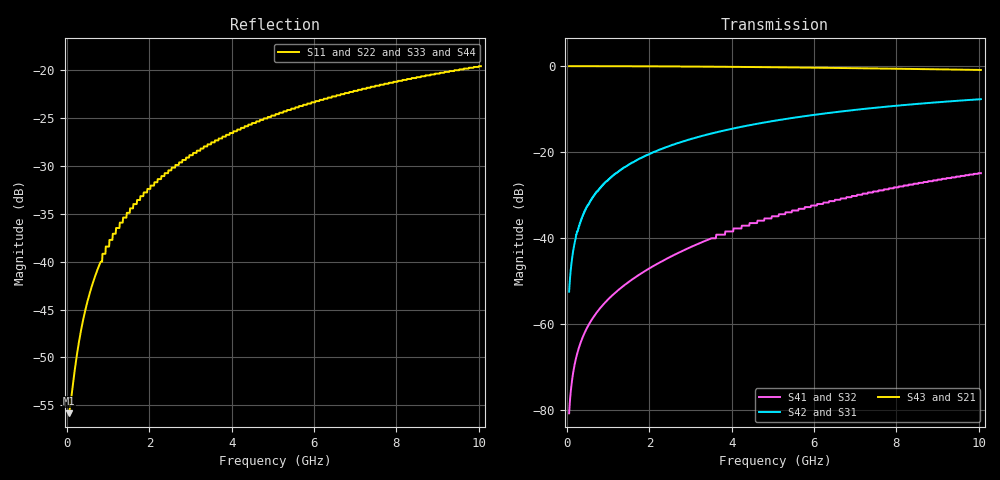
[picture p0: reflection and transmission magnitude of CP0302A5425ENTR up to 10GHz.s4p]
!	AVX THIN FILM OPERATION
!	CP0302A5425ENTR HIGH DIRECTIVITY  COUPLER
!	P/N's CP0302A5425ENTR
! 	18 August 2013
# MHZ S MA R 50
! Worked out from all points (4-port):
!   1000 points, 50 MHz to 10.05 GHz, reference 50 ohm
!   strongest paths, dB at 50 MHz, 2.553 GHz, 5.055 GHz, 7.558 GHz, 10.05 GHz:
!     S43: 0.0, -0.1, -0.3, -0.6, -0.9
!     S21: 0.0, -0.1, -0.3, -0.6, -0.9
!     S42: -52.4, -18.3, -12.7, -9.6, -7.7
!     S31: -52.4, -18.3, -12.7, -9.6, -7.7
!     S41: -80.7, -44.1, -34.9, -29.1, -24.9
!     S32: -80.7, -44.1, -34.9, -29.1, -24.9
!   lowest |S11| = -55.8 dB at 50 MHz (marker M1), VSWR 1.00, Z = 50.2 + j0.0605 ohm
!   |S11| at or under -10 dB: start of sweep to end of sweep
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50  0.001616 21.9  0.998 -0.2  0.002398 89.8  9.252e-05 90.6
    0.998 -0.2  0.001616 21.9  9.252e-05 90.6  0.002398 89.8
    0.002398 89.8  9.252e-05 90.6  0.001616 21.9  0.998 -0.2
    9.252e-05 90.6  0.002398 89.8  0.998 -0.2  0.001616 21.9
240.19  0.003279 62.1  0.998 -0.9  0.012 89.2  0.0004459 93.4
        0.998 -0.9  0.003279 62.1  0.0004459 93.4  0.012 89.2
        0.012 89.2  0.0004459 93.4  0.003279 62.1  0.998 -0.9
        0.0004459 93.4  0.012 89.2  0.998 -0.9  0.003279 62.1
590.541  0.007322 76.4  0.998 -2.1  0.028 87.9  0.001114 98.3
         0.998 -2.1  0.007322 76.4  0.001114 98.3  0.028 87.9
         0.028 87.9  0.001114 98.3  0.007322 76.4  0.998 -2.1
         0.001114 98.3  0.028 87.9  0.998 -2.1  0.007322 76.4
1131.081  0.014 80.2  0.997 -4.0  0.054 86.0  0.002243 105.2
          0.997 -4.0  0.014 80.2  0.002243 105.2  0.054 86.0
          0.054 86.0  0.002243 105.2  0.014 80.2  0.997 -4.0
          0.002243 105.2  0.054 86.0  0.997 -4.0  0.014 80.2
2062.012  0.025 80.2  0.993 -7.3  0.098 82.8  0.004656 114.2
          0.993 -7.3  0.025 80.2  0.004656 114.2  0.098 82.8
          0.098 82.8  0.004656 114.2  0.025 80.2  0.993 -7.3
          0.004656 114.2  0.098 82.8  0.993 -7.3  0.025 80.2
5355.305  0.062 73.0  0.966 -18.6  0.245 71.6  0.02 122.8
          0.966 -18.6  0.062 73.0  0.02 122.8  0.245 71.6
          0.245 71.6  0.02 122.8  0.062 73.0  0.966 -18.6
          0.02 122.8  0.245 71.6  0.966 -18.6  0.062 73.0
10050  0.105 64.0  0.901 -33.3  0.413 57.4  0.057 112.8
       0.901 -33.3  0.105 64.0  0.057 112.8  0.413 57.4
       0.413 57.4  0.057 112.8  0.105 64.0  0.901 -33.3
       0.057 112.8  0.413 57.4  0.901 -33.3  0.105 64.0
